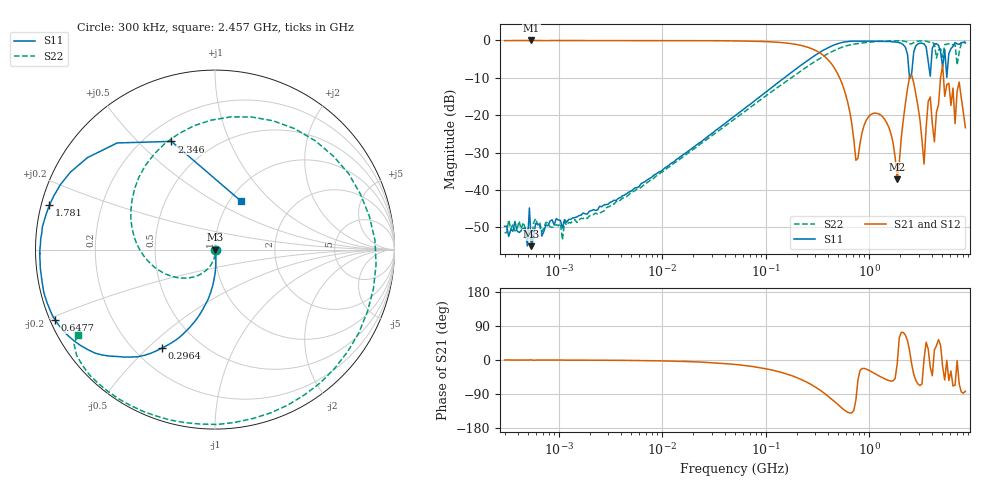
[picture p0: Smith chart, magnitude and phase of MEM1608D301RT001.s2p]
! S-Parameter Data Generated by TDK Corporation
! Copyright(C) 2025 TDK Corporation.
! All Rights Reserved.
! TDK P/N: MEM1608D301RT001 (3-terminal Filter)
! Property: Fc=300MHz
! Size(LxWxT): 1.6x0.8x0.6mm
! Model Type: s2p (Touchstone File Format Version 1.0)
! Frequency: DC=Yes Start=0.3MHz Stop=8500MHz 225points Log-sweep
! Model Generated on Feb. 6, 2025
! Terms and conditions regarding TDK Simulation Models:
! 1)This simulation model is being provided solely for informational
!  purposes. Please refer to the specifications of the products in
!  terms of detailed characteristics of such products.
! 2)In no event shall TDK Corporation of any of its subsidiaries be
!  liable for any loss or damage arising, directly or indirectly,
!  from any information contained in this simulation model, including,
!  but not limited to loss or damages arising from any inaccuracies,
!  omissions or errors in connection with such information.
! 3)Any and all copyrights on this simulation model are owned by
!  TDK Corporation.  Duplication or redistribution of this simulation
!  model without prior written permission from TDK Corporation
!  is prohibited.
! 4)This simulation model is subject to any modification or change
!  without any prior notice.
! 5)Neither TDK Corporation nor any of its subsidiaries shall make any
!  warranty, express or implied, including but not limited to the
!  correctness, implied warranties of merchantability and fitness for
!  a particular purpose with respect to this simulation models.
! 6)The use of this simulation model shall be deemed to have consented
!  to the terms and conditions hereof.
! Port Assignments:
!  1 ---@@@--- 2
! Applicable Conditions:
!  Temperature = 25 degC
!  DC Bias Current = 0 A
!  DC Bias Voltage = 0 V
!  Small Signal Operation
# Hz S MA R 50
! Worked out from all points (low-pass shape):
!   224 points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, 300 kHz to 8.5 GHz, reference 50 ohm
!   highest |S21| = 0.00 dB at 545.3 kHz (marker M1); lowest = -37.1 dB at 1.864 GHz (marker M2)
!   |S21| within 3 dB of the highest: start of sweep to 318.8 MHz
!   lowest |S11| = -55.0 dB at 545.3 kHz (marker M3), VSWR 1.00, Z = 49.8 - j0.0703 ohm
!   |S11| at or under -10 dB: start of sweep to 151.1 MHz; 2.452 GHz to 2.479 GHz (26.68 MHz wide, 1.08 % of centre)
!   |S22| runs from -55.0 to -0.1 dB; largest |S21 - S12| = 0.0079
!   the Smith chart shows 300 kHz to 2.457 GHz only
!   S11 on the Smith chart (normalised r, x): 300 kHz: 1.01, -0.00; 296.4 MHz: 0.31, -0.55; 647.7 MHz: 0.01, -0.21; 1.781 GHz: 0.02, +0.13; 2.346 GHz: 0.30, +0.63; 2.457 GHz: 1.13, +0.67
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300000  0.003275 -9.9  0.9941 -0.1  0.9939 -0.1  0.002709 -6.6
545346.1  0.001776 -156.6  1 0.4  1 0.2  0.001776 -22.8
1721110  0.004926 -39.7  0.997 -0.4  0.9959 -0.4  0.004152 -49.4
9430415  0.01759 -78.3  0.9968 -2.2  0.996 -2.2  0.01656 -83.0
5.167171e7  0.101 -87.8  0.9861 -12.0  0.9846 -12.0  0.09181 -105.6
2.831228e8  0.5989 -116.7  0.7688 -66.9  0.7687 -66.8  0.4988 160.1
2.964424e8  0.6251 -118.4  0.747 -70.2  0.7466 -70.2  0.519 154.5
6.47669e8  0.9732 -156.1  0.1129 -140.0  0.1129 -140.0  0.8671 20.9
7.434462e8  0.9816 -162.6  0.02501 -105.9  0.02495 -106.1  0.9013 -5.4
1.551304e9  0.9705 172.6  0.06843 -54.4  0.0684 -54.4  0.9835 -109.7
1.78071e9  0.9552 165.0  0.02743 -48.4  0.02748 -48.1  0.9897 -122.8
1.864484e9  0.9464 161.5  0.01395 -10.5  0.01398 -10.5  0.9897 -127.0
2.346313e9  0.65 112.0  0.2278 50.8  0.2278 50.8  0.9453 -146.2
2.456696e9  0.3061 61.4  0.3264 24.4  0.3262 24.5  0.9024 -148.1
2.693286e9  0.701 -137.0  0.2696 -37.8  0.2702 -37.9  0.9385 -148.3
3.389298e9  0.9008 157.4  0.02222 3.4  0.02225 3.4  0.9825 -163.7
3.7157e9  0.5171 107.8  0.153 29.0  0.153 29.0  0.9569 -170.6
4.265177e9  0.8914 -179.4  0.04416 26.6  0.0441 26.5  0.8978 173.6
5.126239e9  0.4401 167.6  0.467 -18.6  0.4665 -18.5  0.5951 -164.0
5.884306e9  0.6681 -146.7  0.2684 -54.4  0.2684 -54.5  0.9049 -179.4
7.072242e9  0.8991 163.1  0.2107 -1.5  0.2109 -1.4  0.4713 133.1
8.5e9  0.9284 142.2  0.068 -82.0  0.0682 -82.1  0.9739 176.9
